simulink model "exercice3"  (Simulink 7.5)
settings: Solver=ode45  StartTime=0.0  StopTime=10.0  RelTol=1e-3

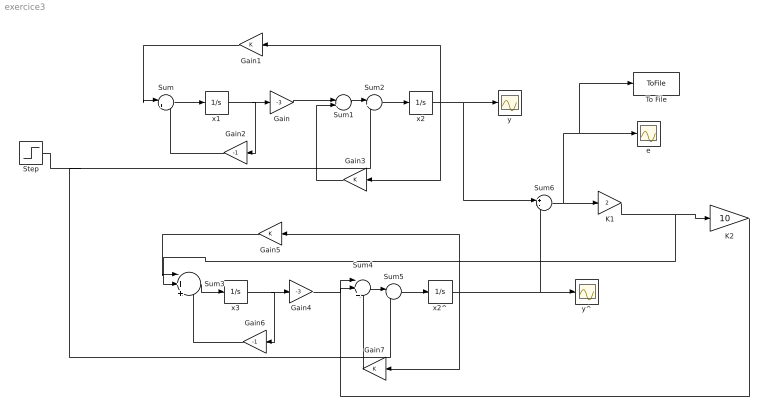
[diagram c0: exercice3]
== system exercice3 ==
  Gain : Gain  Gain=-3
  Gain{1,3,5,7} (4 alike) : Gain
  Gain2 : Gain  Gain=-1
  Gain4 : Gain  Gain=-3
  Gain6 : Gain  Gain=-1
  K1 : Gain  Gain=2
  K2 : Gain  Gain=10
  Step : Step  SampleTime=0
  Sum{,1..2,5} (4 alike) : Sum  Inputs=|++
  Sum3 : Sum  Inputs=|+++
  Sum4 : Sum  Inputs=|+++
  Sum6 : Sum  Inputs=+-
  To File : ToFile  Filename=eluenberger.mat
  e : Scope
  x1 : Integrator  InitialCondition=1
  x2 : Integrator  InitialCondition=1
  x2^ : Integrator  InitialCondition=1
  x3 : Integrator  InitialCondition=10
  y : Scope
  y^ : Scope
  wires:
  Gain/1 -> Sum1/1
  Sum/1 -> x1/1
  x1/1 -> Gain/1, Gain2/1
  Gain2/1 -> Sum/2
  x2/1 -> Gain3/1, Gain1/1, y/1, Sum6/1
  Gain3/1 -> Sum1/2
  Gain1/1 -> Sum/1
  Sum1/1 -> Sum2/1
  Sum2/1 -> x2/1
  Step/1 -> Sum2/2, Sum5/2
  Gain4/1 -> Sum4/1
  Sum3/1 -> x3/1
  x3/1 -> Gain4/1, Gain6/1
  x2^/1 -> Gain7/1, Gain5/1, Sum6/2, y^/1
  Gain5/1 -> Sum3/1
  Sum4/1 -> Sum5/1
  Sum5/1 -> x2^/1
  Sum6/1 -> K1/1, e/1, To File/1
  Gain6/1 -> Sum3/3
  K1/1 -> Sum3/2, K2/1
  Gain7/1 -> Sum4/3
  K2/1 -> Sum4/2
